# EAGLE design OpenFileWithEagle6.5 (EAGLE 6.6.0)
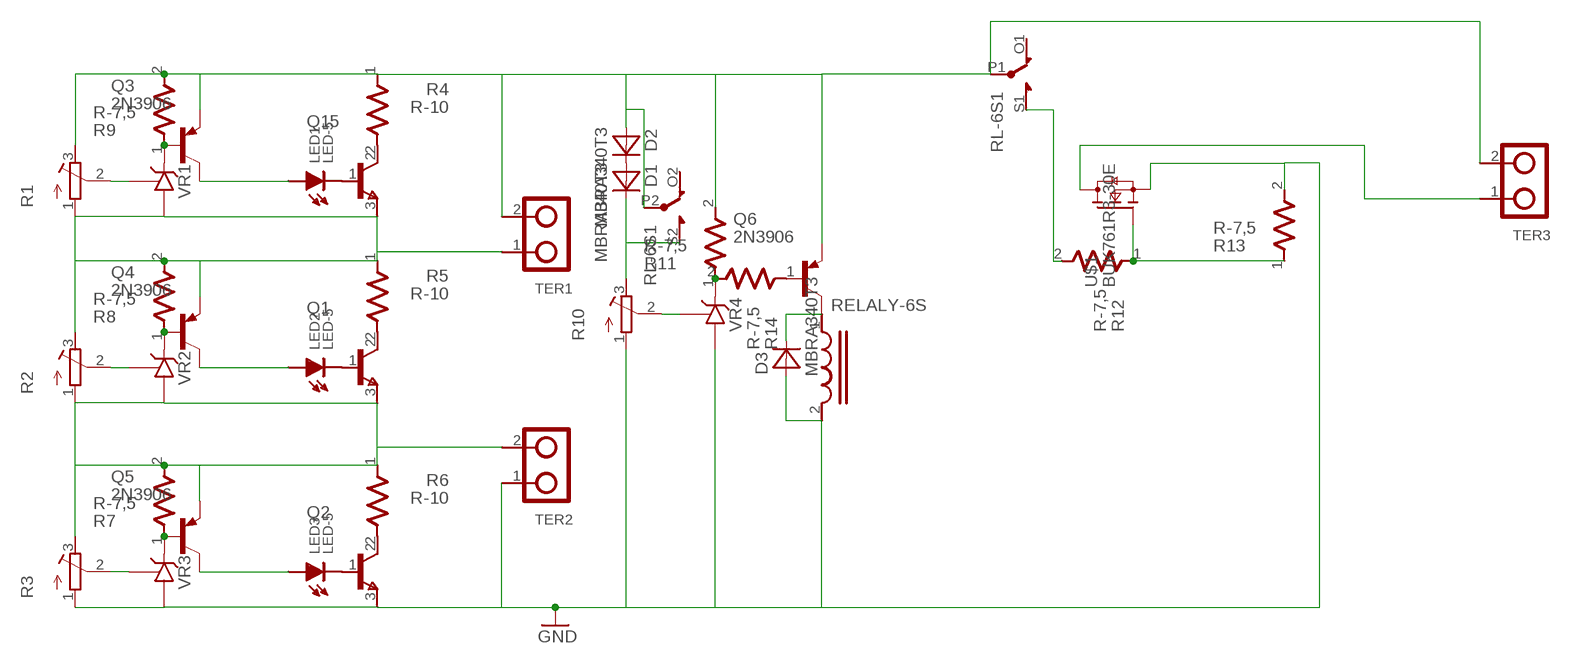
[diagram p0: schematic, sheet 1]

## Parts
D1  MBRA340T3  [SMA]
D2  MBRA340T3  [SMA]
D3  MBRA340T3  [SMA]
LED1  LED-5  [LED5]
LED2  LED-5  [LED5]
LED3  LED-5  [LED5]
Q1  C1815  [TO92L]
Q2  C1815  [TO92L]
Q3  2N3906  [TO92]
Q4  2N3906  [TO92]
Q5  2N3906  [TO92]
Q6  2N3906  [TO92]
Q15  C1815  [TO92L]
R1  R-TRIMM64W  [RTRIM64W]
R2  R-TRIMM64W  [RTRIM64W]
R3  R-TRIMM64W  [RTRIM64W]
R4  R-10  [R-10]
R5  R-10  [R-10]
R6  R-10  [R-10]
R7  R-7,5  [R-7,5]
R8  R-7,5  [R-7,5]
R9  R-7,5  [R-7,5]
R10  R-TRIMM64W  [RTRIM64W]
R11  R-7,5  [R-7,5]
R12  R-7,5  [R-7,5]
R13  R-7,5  [R-7,5]
R14  R-7,5  [R-7,5]
RL-6S1  RELALY-6S  [RELAY-6S]
TER1  DOMINO-2  [DOMI-2]
TER2  DOMINO-2  [DOMI-2]
TER3  DOMINO-2  [DOMI-2]
U$1  BUK761R3-30E  [SOT404]
VR1  TL431CLP  [TO92-CLP]
VR2  TL431CLP  [TO92-CLP]
VR3  TL431CLP  [TO92-CLP]
VR4  TL431CLP  [TO92-CLP]

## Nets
GND: D3.A Q2.3(E) R3.1(A) R10.1(A) R13.2 RL-6S1.2 TER2.1 U$1.3(S) VR3.A VR4.A
N$1: LED1.K Q15.1(B)
N$2: LED2.K Q1.1(B)
N$3: LED3.K Q2.1(B)
N$4: R10.2(S) VR4.R
N$5: R11.1 R14.2 VR4.C
N$6: Q6.2(B) R14.1
N$7: R2.2(S) VR2.R
N$8: R3.2(S) VR3.R
N$9: Q3.2(B) R9.1 VR1.C
N$10: Q4.2(B) R8.1 VR2.C
N$11: Q5.2(B) R7.1 VR3.C
N$12: LED2.A Q4.1(C)
N$13: LED3.A Q5.1(C)
N$14: LED1.A Q3.1(C)
N$15: Q15.2(C) R4.2
N$16: Q1.2(C) R5.2
N$17: Q2.2(C) R6.2
N$18: Q1.3(E) Q5.3(E) R2.1(A) R3.3(E) R6.1 R7.2 TER2.2 VR2.A
N$19: Q4.3(E) Q15.3(E) R1.1(A) R2.3(E) R5.1 R8.2 TER1.1 VR1.A
N$20: D2.A Q3.3(E) Q6.3(E) R1.3(E) R4.1 R9.2 R11.2 RL-6S1.P1(P) RL-6S1.P2(K:P) TER1.2 TER3.2
N$21: R1.2(S) VR1.R
N$22: D3.C Q6.1(C) RL-6S1.1
N$23: TER3.1 U$1.MB(D)
N$25: D1.C R10.3(E) RL-6S1.S2(K:S)
N$26: R12.1 R13.1 U$1.1(G)
N$27: D1.A D2.C
N$28: R12.2 RL-6S1.S1(S)
Unconnected: RL-6S1.O1(O) RL-6S1.O2(K:O)

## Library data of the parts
D1-D3 = diode:MBRA340T3: Surface Mount Schottky Power Rectifier
LED1-LED3 = chuong:LED-5
Q1 Q2 Q15 = lbr:C1815
Q3-Q6 = lbr:2N3906: PNP Transistor
R1-R3 R10 = chuong:R-TRIMM: Trimm resistor
R4-R6 = lbr:R-10
R7-R9 R11-R14 = chuong:R-7,5
RL-6S1 = chuong:RELALY-6S
TER1-TER3 = chuong:DOMINO-2
U$1 = lbr:BUK761R3-30E: N-channel TrenchMOS standard level FET Standard level N-channel MOSFET in a SOT404 package using TrenchMOS technology. This product has been designed and qualified to AEC Q101 standard for use in high performance automotive applications. AAL Eindhoven MK
VR1-VR4 = chuong:TL431CLP: VOLTAGE REGULATOR

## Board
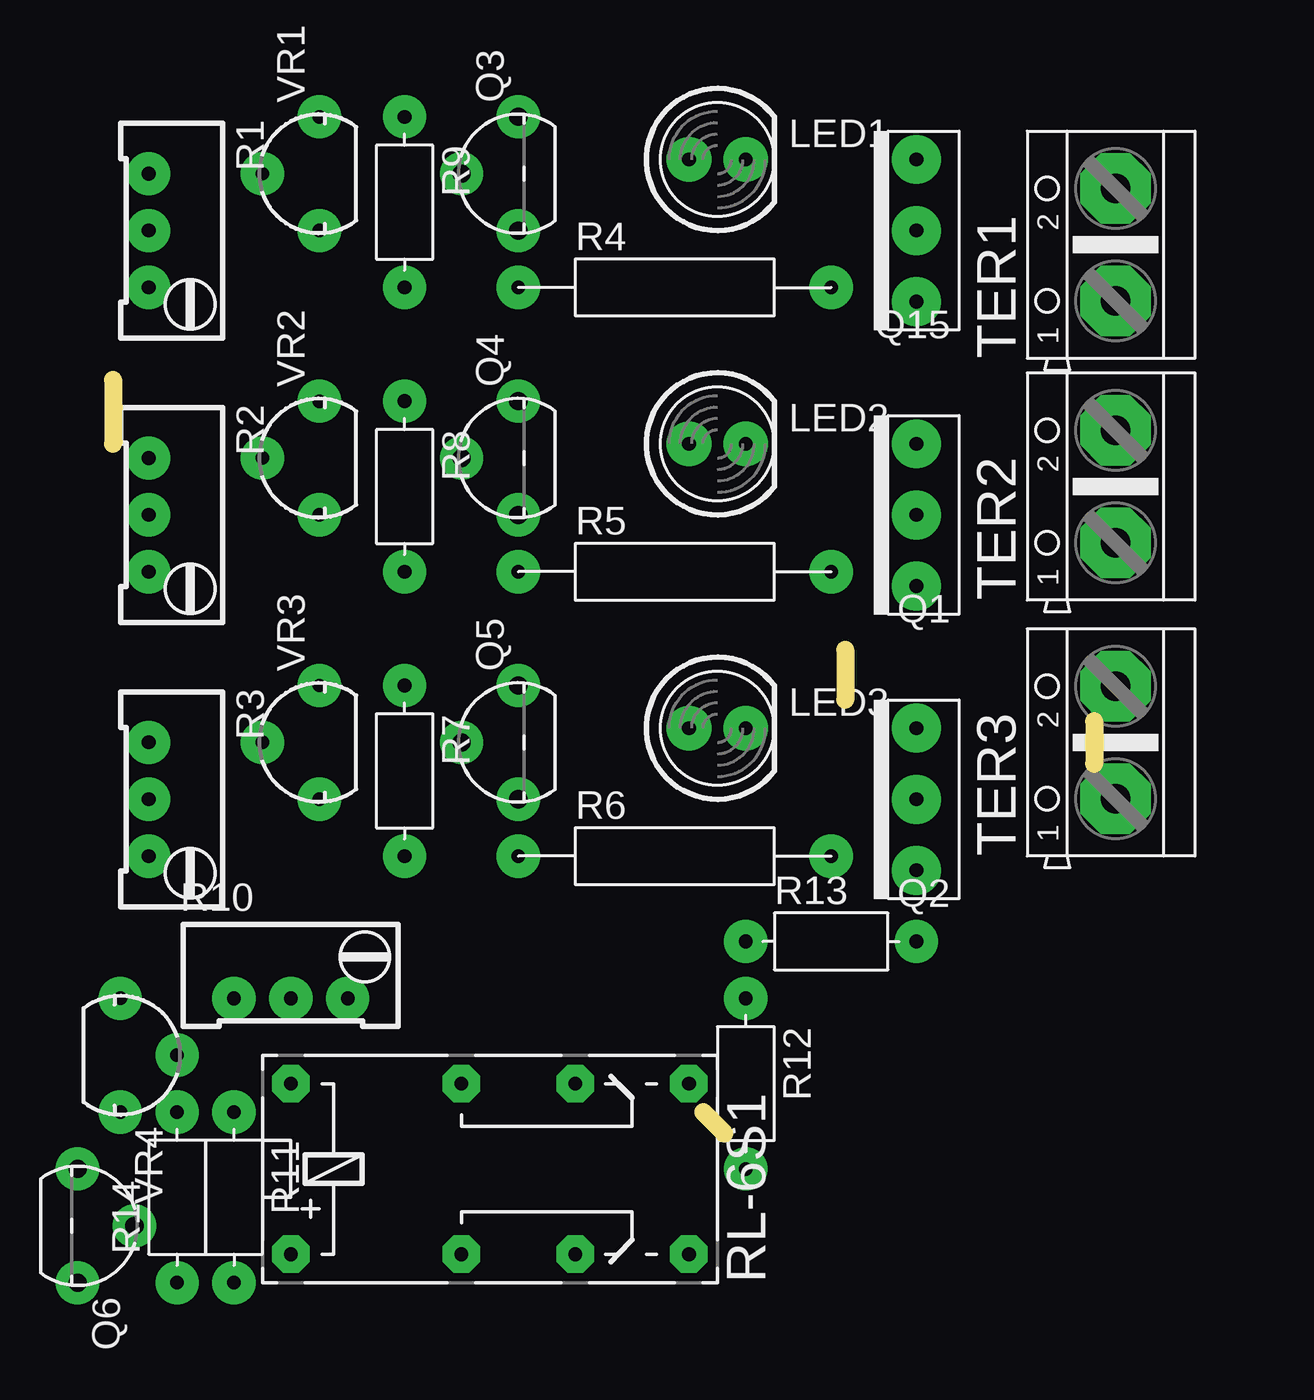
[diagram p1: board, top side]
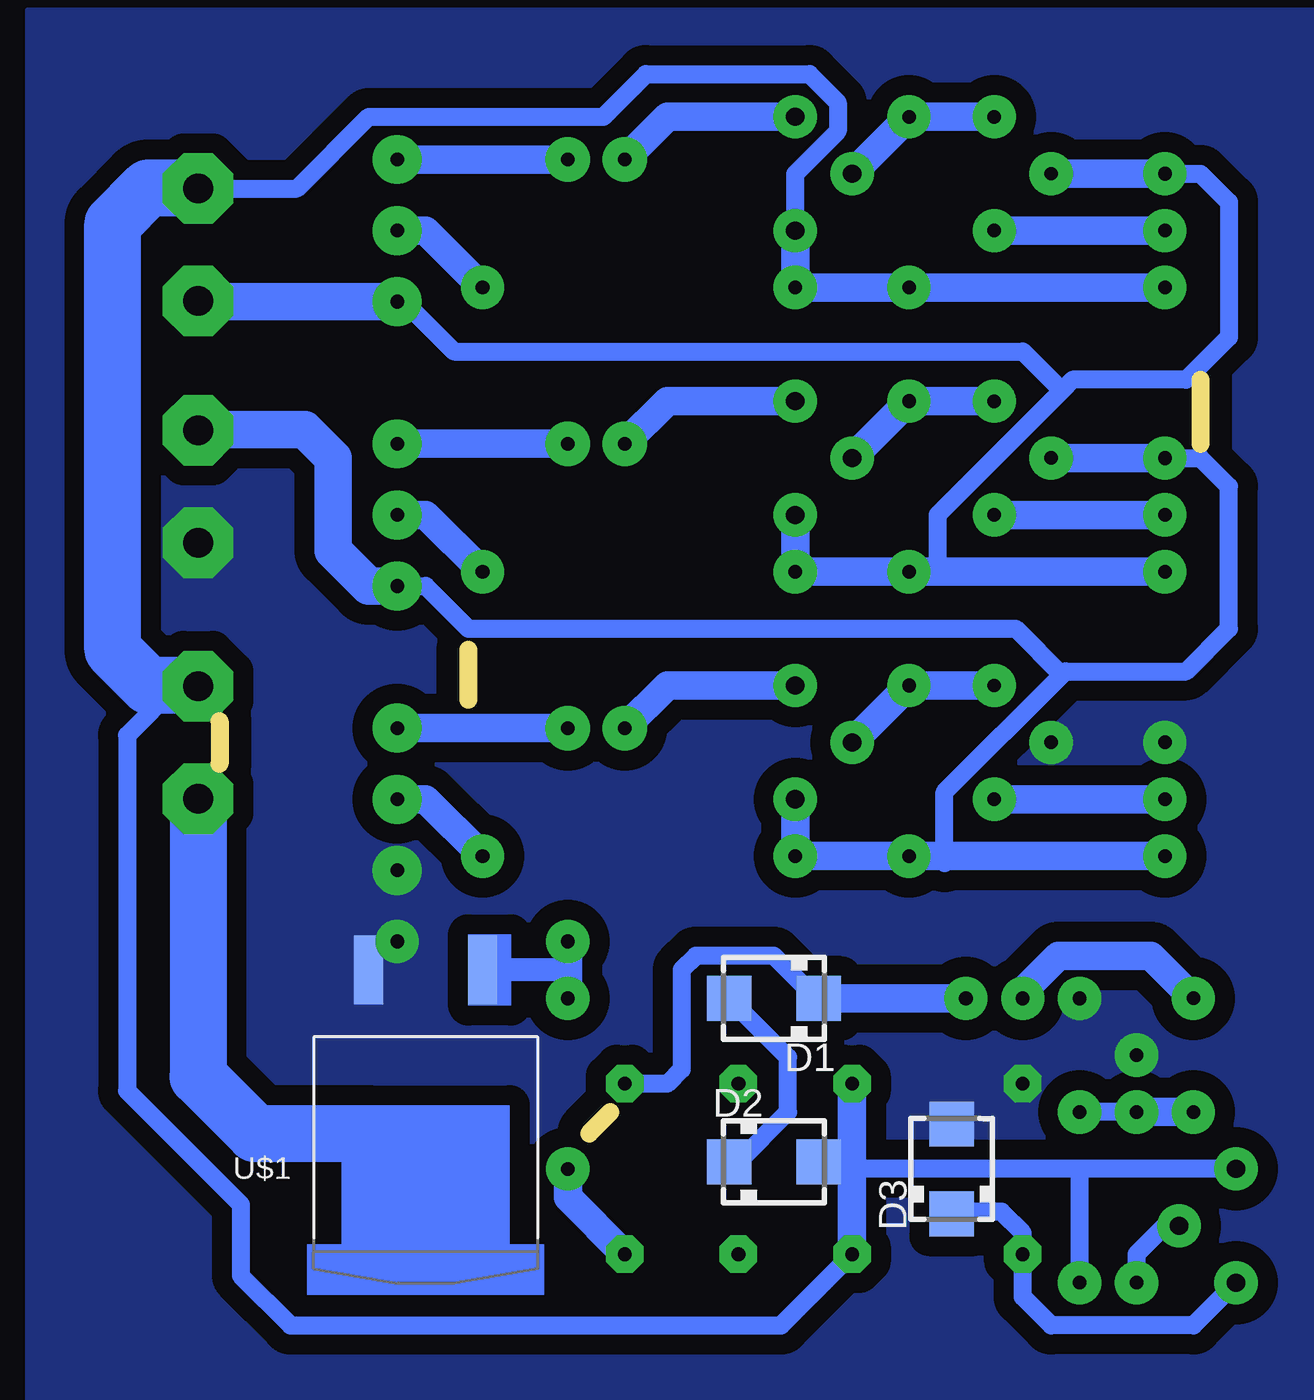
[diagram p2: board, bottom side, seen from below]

Size 43.81 x 33.66 mm. Coordinates in mm from the lower left corner, seen from the top.
Outline: 26.35,0.95 27.3,0
Outline: 32.7,21.59 32.7,19.37
Outline: 0,33.66 0,30.8
Outline: 43.82,18.41 43.82,16.51
Copper layers (1*16): Top 0.035mm / dielectric 1.5mm / Bottom 0.035mm
Design rules "default": minimum track width 10mil, minimum drill 24mil, track to track 8mil, track to pad 8mil, pad to pad 8mil, via to via 8mil, smd to smd 8mil, copper to edge 40mil, drill to drill 8mil, minimum pad ring 10mil, minimum via ring 8mil, stop-mask expansion 4mil, vias tented up to drill 0mil, thermal gap 10mil

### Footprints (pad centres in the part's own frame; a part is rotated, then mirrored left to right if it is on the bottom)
SMA = smd 2 x 2: A 2,0; C -2,0
LED5 = drill 0.61 pad 2: A -1.27,0; K 1.27,0
TO92L = drill 0.61 pad 2.184: 1 3.175,0; 2 0,0; 3 -3.175,0
TO92 = drill 0.813 pad 1.93: 1 2.54,0; 2 0,2.54; 3 -2.54,0
RTRIM64W = drill 0.61 pad 1.93: 1 1.27,-2.54; 2 1.27,0; 3 1.27,2.54
R-10 = drill 0.61 pad 1.93: 1 -7.62,0; 2 6.35,0
R-7,5 = drill 0.61 pad 1.93: 1 -3.81,0; 2 3.81,0
RELAY-6S = drill 0.61 pad 1.676 octagon: 1 -10.16,-3.81; 2 -10.16,3.81; O1 2.54,-3.81; O2 2.54,3.81; P1 -2.54,-3.81; P2 -2.54,3.81; S1 7.62,-3.81; S2 7.62,3.81
DOMI-2 = drill 1.321 pad 3.15 octagon: 1 -2.515,0; 2 2.515,0
SOT404 = smd 1.3 x 3.1: 1 -2.54,-6.35; 3 2.54,-6.35 | smd 0 x 0: MB 0,0
TO92-CLP = drill 0.6 pad 1.93: A 0,2.54; C 2.54,0; R -2.54,0

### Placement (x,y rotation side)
D1  19.05,6.03 180 bottom
D2  19.05,-1.27 0 bottom
D3  11.11,-1.59 90 bottom
LED1  26.99,43.5 0 top  (outside the outline)
LED2  26.99,30.8 0 top
LED3  26.99,18.1 0 top
Q1  35.88,27.62 90 top
Q2  35.88,14.92 90 top
Q3  18.1,42.86 90 top  (outside the outline)
Q4  18.1,30.16 90 top
Q5  18.1,17.46 90 top
Q6  -1.59,-4.13 270 top
Q15  35.88,40.32 90 top  (outside the outline)
R1  2.86,40.32 180 top  (outside the outline)
R2  2.86,27.62 180 top
R3  2.86,14.92 180 top
R4  25.72,37.78 0 top  (outside the outline)
R5  25.72,25.08 0 top
R6  25.72,12.38 0 top
R7  13.02,16.19 270 top
R8  13.02,28.89 270 top
R9  13.02,41.59 270 top  (outside the outline)
R10  7.94,7.3 270 top
R11  5.4,-2.86 270 top
R12  28.26,2.22 270 top
R13  32.07,8.57 0 top
R14  2.86,-2.86 90 top
RL-6S1  18.1,-1.59 0 top
TER1  44.77,39.69 90 top  (outside the outline)
TER2  44.77,28.89 90 top
TER3  44.77,17.46 90 top
U$1  34.61,0.95 180 bottom
VR1  9.21,42.86 90 top  (outside the outline)
VR2  9.21,30.16 90 top
VR3  9.21,17.46 90 top
VR4  0.32,3.49 270 top

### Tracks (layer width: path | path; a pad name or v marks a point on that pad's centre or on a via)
GND
  pour Bottom (isolate 0.889, no thermals): -5.08,50.16 52.39,50.16 52.39,-12.07 -5.08,-12.07
N$1
  Bottom 1.27: LED1.K Q15.1
N$2
  Bottom 1.27: LED2.K Q1.1
N$3
  Bottom 1.27: LED3.K Q2.1
N$4
  Bottom 1.27: R10.2 7.94,6.35 6.35,7.94 2.22,7.94 VR4.R
N$5
  Bottom 0.813: R14.2 R11.1
  Bottom 1.27: VR4.C R14.2
N$6
  Bottom 0.813: Q6.2 1.59,-4.13 2.86,-5.4 R14.1
N$7
  Bottom 1.27: R2.2 VR2.R
N$8
  Bottom 1.27: VR3.R R3.2
N$9
  Bottom 1.27: VR1.C R9.1 Q3.2
N$10
  Bottom 1.27: VR2.C R8.1 Q4.2
N$11
  Bottom 1.27: VR3.C R7.1 Q5.2
N$12
  Bottom 1.27: Q4.1 23.81,32.7 LED2.A
N$13
  Bottom 1.27: Q5.1 23.81,20 LED3.A
N$14
  Bottom 1.27: Q3.1 23.81,45.4 LED1.A
N$15
  Bottom 1.27: Q15.2 34.61,40.32 R4.2
N$16
  Bottom 1.27: Q1.2 34.61,27.62 R5.2
N$17
  Bottom 1.27: Q2.2 34.61,14.92 R6.2
N$18
  Bottom 0.813: R2.1 0,30.16 -1.27,28.89 -1.27,22.54 0.63,20.64 6.03,20.64 6.19,20.48 | Q1.3 34.61,24.45 32.7,22.54 8.26,22.54 6.19,20.48 | R3.3 11.11,12.38 11.43,12.07 11.43,15.24 6.19,20.48
  Bottom 1.27: R2.1 VR2.A | R3.3 R7.2 R6.1 Q5.3
  Bottom 1.676: TER2.2 44.74,31.43 40,31.43 38.74,30.16 38.74,26.03 37.15,24.45 Q1.3
N$19
  Bottom 0.813: R1.1 0,42.86 -1.27,41.59 -1.27,35.56 0.63,33.66 5.71,33.66 6.19,33.18 | 6.19,33.18 11.75,27.62 11.75,25.4 12.07,25.08 | Q15.3 35.56,37.15 33.34,34.92 7.94,34.92 6.19,33.18
  Bottom 1.27: R1.1 VR1.A | R2.3 12.07,25.08 R8.2 R5.1 Q4.3
  Bottom 1.676: Q15.3 44.74,37.15 TER1.1
N$20
  Bottom 0.813: Q3.3 18.1,42.86 16.19,44.77 16.19,46.04 17.46,47.31 24.76,47.31 26.67,45.4 37.15,45.4 40.35,42.2 TER1.2 | TER3.2 45.75,19.98 47.94,17.78 47.94,1.9 42.86,-3.17 42.86,-6.35 40.64,-8.57 18.73,-8.57 RL-6S1.P1 | Q6.3 5.4,-1.59 | 5.4,-1.59 15.24,-1.59 15.56,-1.91 | R11.2 5.4,-1.59
  Bottom 1.27: R1.3 R9.2 R4.1 Q3.3 | RL-6S1.P2 15.56,-1.27 | D2.A 15.56,-1.27 | RL-6S1.P1 15.56,-1.91 15.56,-1.27
  Bottom 2.54: TER3.2 44.79,20 46.99,20 48.58,21.59 48.58,40.64 46.99,42.23 44.79,42.23 TER1.2
N$21
  Bottom 1.27: R1.2 VR1.R
N$22
  Bottom 0.813: D3.C 11.02,-3.49 8.89,-3.49 7.94,-4.44 RL-6S1.1 7.94,-7.3 6.67,-8.57 0.32,-8.57 Q6.1
N$23
  Bottom 0.254: U$1.MB 36.2,0.95 37.15,0
  Bottom 2.54: TER3.1 44.77,2.54 42.23,0 37.15,0 34.61,-2.54
N$25
  Bottom 0.813: 17.05,6.26 17.37,6.26 19.05,7.94 22.54,7.94 23.18,7.3 23.18,2.86 23.81,2.22 RL-6S1.S2
  Bottom 1.27: R10.3 D1.C 17.05,6.26
N$26
  Bottom 1.016: 28.26,7.3 U$1.1
  Bottom 1.27: R13.1 28.26,7.3 R12.1
N$27
  Bottom 0.813: 21.27,-1.27 20.64,-1.27 18.41,0.95 18.41,3.4 D1.A
  Bottom 1.27: D2.C 21.27,-1.27
N$28
  Bottom 1.27: R12.2 28.26,-2.86 RL-6S1.S1
(copper drawn outside any net)
  shapes: Bottom area x1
